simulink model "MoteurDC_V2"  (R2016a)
settings: Solver=ode15s  StartTime=0.0  StopTime=3600  RelTol=1e-3
libraries: fl_lib x11, nesl_utility x5, elec_lib x2

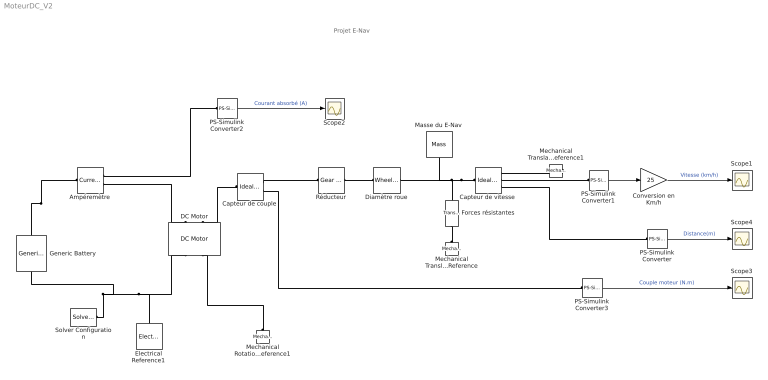
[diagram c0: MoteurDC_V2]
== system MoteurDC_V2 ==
  note: Projet E-Nav
  Ampéremètre : fl_lib/Electrical/Electrical Sensors/Current Sensor
  Capteur de couple : fl_lib/Mechanical/Mechanical Sensors/Ideal Torque Sensor
  Capteur de vitesse : fl_lib/Mechanical/Mechanical Sensors/Ideal Translational Motion Sensor  offset=0 m
  Conversion en Km/h : Gain  Gain=25
  DC Motor : elec_lib/Actuators & Drivers/Rotational Actuators/DC Motor  parameterization=1  Ra=3.9 Ohm  La=0 H  emf_or_torque=1  Kv=0.4 V/(rad/s)  Ki=6.876e-4 N*m/A  T_stall=2.4e-4 N*m  w_max=1.91e+4 rpm  w_rated=1.5e+4 rpm  P_rated=0.08 W  V_rated=1.5 V  J=0.01 kg*m^2  lam_param=2  lam=0 N*m/(rad/s)  i_noload=0 A  V_i_noload=1.5 V  speed0=0 rpm  alpha=0.00393 1/K  Tmeas=25 C  thermal_mass=100 J/K  initial_temperature=25 C
  Diamètre roue : fl_lib/Mechanical/Mechanisms/Wheel and Axle  R=57.14 cm  or=1  t_specify=off  t_priority=High  t=0 N*m  f_specify=off  f_priority=High  f=0 N
  Electrical Reference1 : fl_lib/Electrical/Electrical Elements/Electrical Reference
  Forces résistantes : fl_lib/Mechanical/Translational Elements/Translational Friction  brkwy_frc=25 N  Col_frc=20 N  visc_coef=100 N/(m/s)  trans_coef=10 s/m  vel_thr=1e-4 m/s  v_specify=off  v_priority=High  v=0 m/s  f_specify=off  f_priority=High  f=0 N
  Generic Battery : elec_lib/Sources/Generic Battery  Vnom=200 V  R1=2 Ohm  prm_AH=1  AH=50 hr*A  AH0=50 hr*A  V1=11.5 V  AH1=25 hr*A  prm_R2=1  R2=2e+3 Ohm
  Masse du E-Nav : fl_lib/Mechanical/Translational Elements/Mass  mass=20000 kg  v_specify=off  v_priority=High  v=0 m/s  f_specify=off  f_priority=High  f=0 N
  Mechanical Rotational Reference1 : fl_lib/Mechanical/Rotational Elements/Mechanical Rotational Reference
  Mechanical Translational Reference : fl_lib/Mechanical/Translational Elements/Mechanical Translational Reference
  Mechanical Translational Reference1 : fl_lib/Mechanical/Translational Elements/Mechanical Translational Reference
  PS-Simulink Converter : nesl_utility/PS-Simulink Converter  PhysicalDomain=network_engine_domain  SubClassName=ps_output  LeftPortType=input  RightPortType=output  PseudoPeriodic=off  Frequencies=[]  Unit=1  AffineConversion=off
  PS-Simulink Converter1 : nesl_utility/PS-Simulink Converter  PhysicalDomain=network_engine_domain  SubClassName=ps_output  LeftPortType=input  RightPortType=output  PseudoPeriodic=off  Frequencies=[]  Unit=1  AffineConversion=off
  PS-Simulink Converter2 : nesl_utility/PS-Simulink Converter  PhysicalDomain=network_engine_domain  SubClassName=ps_output  LeftPortType=input  RightPortType=output  PseudoPeriodic=off  Frequencies=[]  Unit=A  AffineConversion=off
  PS-Simulink Converter3 : nesl_utility/PS-Simulink Converter  PhysicalDomain=network_engine_domain  SubClassName=ps_output  LeftPortType=input  RightPortType=output  PseudoPeriodic=off  Frequencies=[]  Unit=1  AffineConversion=off
  Réducteur : fl_lib/Mechanical/Mechanisms/Gear Box  ratio=6  t_in_specify=off  t_in_priority=High  t_in=0 N*m  t_out_specify=off  t_out_priority=High  t_out=0 N*m
  Scope{1..4} (4 alike) : Scope
  Solver Configuration : nesl_utility/Solver Configuration  PhysicalDomain=network_engine_domain  SubClassName=solver  LeftPortType=input  RightPortType=generic  Accelerate=off  Tones=[]  Harmonics=[]  SimulateNoise=off  Profile=off  UseLocalSampling=off  EnableSwitchedLinearOptims=on  FrequencyDomain=off  UseCCode=off  RelTol=0.001  AbsTol=1e-06  MinStep=1e-09  ToWorkspace=off  RevertToSquareIcSolve=off  NumHomotopyIterations=100  PhasorMode=off  PhasorModeNumHarmonics=1  OverrideAbsTol=off  DoDC=off  ResidualTolerance=1e-09  UseLocalSolver=off  LocalSolverChoice=NE_BACKWARD_EULER_ADVANCER  LocalSolverSampleTime=0.001  DoFixedCost=off  MaxNonlinIter=3  MaxModeIter=2  LinearAlgebra=Sparse  DelaysMemoryBudget=1024  AutomaticFiltering=on  FilteringTimeConstant=0.001
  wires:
  PS-Simulink Converter2/1 -> Scope2/1  "Courant absorbé (A)"
  PS-Simulink Converter3/1 -> Scope3/1  "Couple moteur (N.m)"
  PS-Simulink Converter1/1 -> Conversion en Km/h/1
  Conversion en Km/h/1 -> Scope1/1  "Vitesse (km/h)"
  PS-Simulink Converter/1 -> Scope4/1  "Distance(m)"
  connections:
  Solver Configuration/RConn1 -- Generic Battery/RConn1 -- Electrical Reference1/LConn1 -- DC Motor/RConn1
  Ampéremètre/RConn2 -- DC Motor/LConn1
  PS-Simulink Converter2/LConn1 -- Ampéremètre/RConn1
  Mechanical Rotational Reference1/LConn1 -- DC Motor/RConn2
  Capteur de couple/LConn1 -- DC Motor/LConn2
  Capteur de vitesse/LConn1 -- Masse du E-Nav/LConn1 -- Diamètre roue/RConn1 -- Forces résistantes/LConn1
  Mechanical Translational Reference/LConn1 -- Forces résistantes/RConn1
  Capteur de couple/RConn2 -- PS-Simulink Converter3/LConn1
  PS-Simulink Converter1/LConn1 -- Capteur de vitesse/RConn2
  Mechanical Translational Reference1/LConn1 -- Capteur de vitesse/RConn1
  Réducteur/RConn1 -- Diamètre roue/LConn1
  Capteur de couple/RConn1 -- Réducteur/LConn1
  Ampéremètre/LConn1 -- Generic Battery/LConn1
  Capteur de vitesse/RConn3 -- PS-Simulink Converter/LConn1
